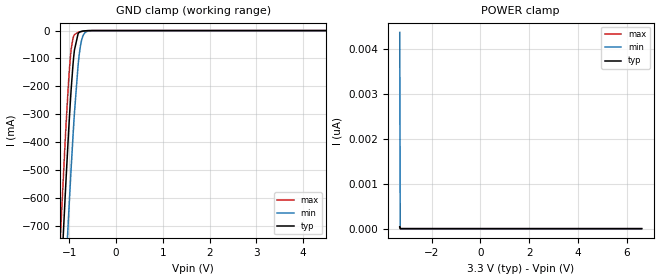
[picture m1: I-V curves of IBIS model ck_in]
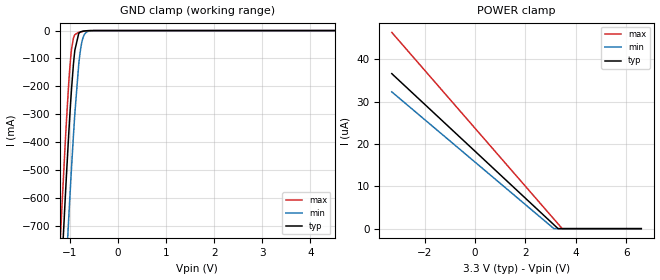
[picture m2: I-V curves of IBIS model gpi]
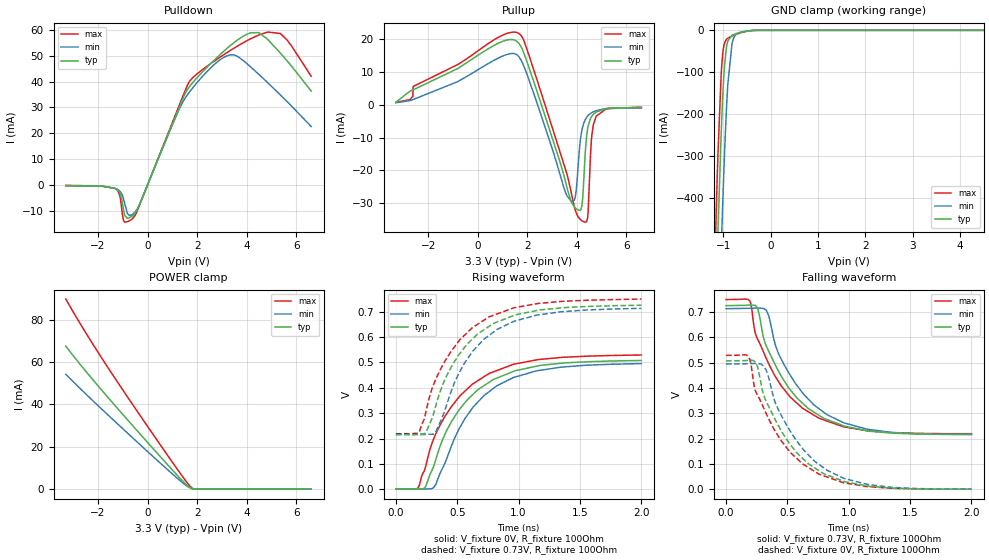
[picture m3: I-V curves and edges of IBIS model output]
|Texas Instruments Incorporated
| Marketing Part # : CDCDB803
| Voltage Range : 3.3V
| Package-type: QFN
| #pins/pkg drawing : 48-pin RSL
[IBIS Ver] 3.2
[File name] cdcdb803.ibs
[File Rev] 1.0
[Date] 07/02/2021
[Source]
| Texas Instruments Incorporated.
| 12500 TI Blvd
| Dallas, TX -75243
[Notes] Revision History:
| Rev 1.0: 07/02/2021
| - Initial version of the model
| - Model generated from simulations in TISPICE/SPECTRE
| - C_comp although listed in numerical order of value are
| obtained from varying PVT conditions. For PVT conditions for
| each specific value refer the buffer description under
| respective [Model]. IBIS model user is responsible for using
| appropriate C_comp to simulate for Signal Integrity.
| - Warnings regarding combined Non-monotonicity of various models have been
| reviewed and considered minor and can be ignored.
[Disclaimer]
| This model is designed as an aid for customers of Texas Instruments.
| TI and its licensors and suppliers make no warranties, either expressed
| or implied, with respect to this model, including the warranties of
| merchantability or fitness for a particular purpose. The model is
| provided solely on an "as is" basis. The entire risk as to its quality
| and performance is with the customer.
| This model is subject to change without notice. Texas Instruments
| Incorporated is not responsible for updating this model.
[Copyright]
(C) Copyright 2021 Texas Instruments Incorporated. All rights reserved.
| Component1 CDCDB803 (per package)
[Component] CDCDB803
[Manufacturer] Texas Instruments Incorporated
[Package] |48 QFN
| variable typ min max
R_pkg 0.111 0.052 0.169
L_pkg 2.02nH 1.12nH 2.9nH
C_pkg 0.163pF 0.062pF 0.264pF
| pin number (pin name) mapping to model name
[Pin] signal_name model_name R_pin L_pin C_pin
1   CLK_IN   ck_in   NA   NA   NA
2   CLK_INz   ck_in   NA   NA   NA
3   CK0P   output   NA   NA   NA
4   CK0N   output   NA   NA   NA
5   CK1P   output   NA   NA   NA
6   CK1N   output   NA   NA   NA
7   CK2P   output   NA   NA   NA
8   CK2N   output   NA   NA   NA
9   CK3P   output   NA   NA   NA
10   CK3N   output   NA   NA   NA
11   CK4P   output   NA   NA   NA
12   CK4N   output   NA   NA   NA
13   CK5P   output   NA   NA   NA
14   CK5N   output   NA   NA   NA
15   CK6P   output   NA   NA   NA
16   CK6N   output   NA   NA   NA
17   CK7P   output   NA   NA   NA
18   CK7N   output   NA   NA   NA
19   POWERGD_POWERDNz   gpi   NA   NA   NA
20   OE0B   gpi   NA   NA   NA
21   OE1B   gpi   NA   NA   NA
22   OE2B   gpi   NA   NA   NA
23   OE3B   gpi   NA   NA   NA
24   OE4B   gpi   NA   NA   NA
25   OE5B   gpi   NA   NA   NA
26   OE6B   gpi   NA   NA   NA
27   OE7B   gpi   NA   NA   NA
28   SMB_WRTLOCK   gpi   NA   NA   NA
29   VDD   POWER   NA   NA   NA
30   VDDR   POWER   NA   NA   NA
31   VDDA   POWER   NA   NA   NA
32   SMBDAT   smbdat   NA   NA   NA
33   SMBCLK   smbclk   NA   NA   NA
34   SADR0   strap_in   NA   NA   NA
35   SADR1   strap_in   NA   NA   NA
[Diff Pin]   inv_pin   vdiff   tdelay_typ  tdelay_min  tdelay_max
1   2   10m   NA   NA   NA
3   4   NA   NA   NA   NA
5   6   NA   NA   NA   NA
7   8   NA   NA   NA   NA
9   10   NA   NA   NA   NA
11   12   NA   NA   NA   NA
13   14   NA   NA   NA   NA
15   16   NA   NA   NA   NA
17   18   NA   NA   NA   NA
| Use Differential pin definition for differential I/Os
|[Diff Pin] inv_pin vdiff tdelay_typ tdelay_min tdelay_max
|3 4 200mV NA NA NA
|15 16 NA NA NA NA
|***** end of component 1 definition
| Models and submodels in the file (6): ck_in (Input), gpi (Input), output (Output), smbclk (Input), smbdat (I/O_open_drain), strap_in (Input)
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| Model Selectors
|***Modify the following as it applies to a speciic model with multiple ****
|*** powver supply options or driver programmability *********
| Model1
|IBIS Model File - Generated by SIMDE
| http://www.iometh.com/Product/SIMDE
[Model]   ck_in
Model_type   Input
Vinl = 0.66
Vinh = 2.64
|   typ   min   max
C_comp   1.16pF   1.09pF   1.19pF
[Voltage Range]   3.3   3.135   3.465
[Temperature Range]   27   125   -40
[Power Clamp Reference]   3.3   3.135   3.465
[GND Clamp Reference]   0   0   0
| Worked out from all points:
|   GND clamp passes 1 mA (typ) near -0.68 V on its own axis
[GND Clamp]
|   Voltage   I(typ)   I(min)   I(max)
-3.3V     -9.039A    -9.284A    -8.888A
-1.191V   -935.5mA   -1.251A    -732mA
-1.162V   -831.2mA   -1.146A    -628.1mA
-1.092V   -595.1mA   -906.9mA   -396mA
-1.023V   -374.9mA   -677.1mA   -191.4mA
-973.5mV  -234.8mA   -521.5mA   -82.42mA
-894.3mV  -70.11mA   -296.5mA   -14.46mA
-815.1mV  -10.89mA   -123.3mA   -6.064mA
-765.6mV  -4.002mA   -55.99mA   -4.283mA
-716.1mV  -1.883mA   -21.3mA    -2.535mA
-557.7mV  -94.7uA    -711uA     -73.04uA
6.6V      0A         0A         0A
[POWER Clamp]
|   Voltage   I(typ)   I(min)   I(max)
-3.3V     45.09pA    4.378nA    27.16pA
-3.28V    0A         0A         0A
-3.27V    0A         0A         0A
6.6V      0A         0A         0A
[Model]   gpi
Model_type   Input
Vinl = 1.2
Vinh = 1.6
|   typ   min   max
C_comp   0.852pF   0.8pF   0.9pF
[Voltage Range]   3.3   3.135   3.465
[Temperature Range]   27   125   -40
[Power Clamp Reference]   3.3   3.135   3.465
[GND Clamp Reference]   0   0   0
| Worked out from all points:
|   GND clamp passes 1 mA (typ) near -0.67 V on its own axis
[GND Clamp]
|   Voltage   I(typ)   I(min)   I(max)
-3.3V     -9.039A    -9.284A    -8.888A
-1.191V   -935.6mA   -1.251A    -732.1mA
-1.162V   -831.3mA   -1.146A    -628.1mA
-1.092V   -595.2mA   -907mA     -396.1mA
-1.023V   -375mA     -677.2mA   -191.6mA
-973.5mV  -235mA     -521.6mA   -82.67mA
-894.3mV  -70.36mA   -296.7mA   -14.69mA
-815.1mV  -11.07mA   -123.5mA   -6.196mA
-765.6mV  -4.101mA   -56.27mA   -4.378mA
-716.1mV  -1.934mA   -21.53mA   -2.594mA
-557.7mV  -100.1uA   -740.4uA   -78.62uA
6.6V      0A         0A         0A
[POWER Clamp]
|   Voltage   I(typ)   I(min)   I(max)
-3.3V     36.61uA    32.31uA    46.35uA
3.125V    960nA      39.57nA    2.319uA
3.293V    26nA       0A         1.165uA
3.462V    0A         0A         11.68nA
6.6V      0A         0A         0A
[Model]   output
Model_type   Output
Polarity   Non-Inverting
Vmeas = 0.365
Vref = 0
Cref = 2pF
Rref = 100000
|   typ   min   max
C_comp   4pF   3.5pF   4.5pF
[Voltage Range]   3.3   3.135   3.465
[Temperature Range]   27   125   -40
[Pullup Reference]   3.3   3.135   3.465
[Pulldown Reference]   0   -0   0
[Power Clamp Reference]   3.3   3.135   3.465
[GND Clamp Reference]   0   0   0
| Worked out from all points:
|   slope of the pulldown table from 0 to 0.495 V, typ, clamps not added: 42.1 ohm
|   GND clamp passes 1 mA (typ) near -0.44 V on its own axis
|   falling waveform, V_fixture 0.73V, R_fixture 100Ohm: 20-80 % time 377ps typ, 384ps min, 383ps max; typ from 0.725 V to 0.217 V
|   rising waveform, V_fixture 0V, R_fixture 100Ohm: 20-80 % time 396ps typ, 395ps min, 402ps max; typ from 0.001 V to 0.508 V
|   rising waveform, V_fixture 0.73V, R_fixture 100Ohm: 20-80 % time 382ps typ, 377ps min, 390ps max; typ from 0.217 V to 0.725 V
|   falling waveform, V_fixture 0V, R_fixture 100Ohm: 20-80 % time 378ps typ, 384ps min, 386ps max; typ from 0.507 V to 0.001 V
[Pulldown]
|   Voltage   I(typ)   I(min)   I(max)
-3.3V     -318.6uA   -393.1uA   -273.4uA
-1.31V    -1.398mA   -1.371mA   -1.435mA
-1.122V   -3.194mA   -2.494mA   -4.283mA
-973.5mV  -9.578mA   -5.349mA   -13.87mA
-815.1mV  -13.03mA   -11.21mA   -14.32mA
-636.9mV  -12.23mA   -11.62mA   -13.37mA
-379.5mV  -8.892mA   -8.671mA   -9.227mA
1.68V     37.96mA    35.85mA    39.95mA
3.244V    53.25mA    50.17mA    51.53mA
4.481V    59.02mA    42.89mA    58.09mA
5.353V    51.13mA    34.87mA    58.68mA
6.6V      36.35mA    22.57mA    42.09mA
[GND Clamp]
|   Voltage   I(typ)   I(min)   I(max)
-3.3V     -10.93A    -11.17A    -10.79A
-1.211V   -881.9mA   -1.2A      -686.4mA
-1.132V   -556.2mA   -867.4mA   -367.4mA
-1.112V   -480.1mA   -787.6mA   -296.1mA
-1.033V   -214.5mA   -487.9mA   -84.47mA
-1.013V   -162.9mA   -419.7mA   -57.48mA
-973.5mV  -85.09mA   -295mA     -30.33mA
-904.2mV  -25.82mA   -129mA     -18.86mA
-815.1mV  -11.68mA   -31.98mA   -13.66mA
-785.4mV  -10.14mA   -20.14mA   -12.18mA
-320.1mV  -99.39uA   -119.7uA   -85.22uA
6.6V      0A         0A         0A
[Pullup]
|   Voltage   I(typ)   I(min)   I(max)
-3.3V     815.4uA    650uA      792.1uA
848.1mV   18.92mA    14.39mA    20.72mA
1.65V     18.91mA    14.82mA    21.89mA
3.759V    -29.34mA   -29.32mA   -26.28mA
3.957V    -31.62mA   -27.07mA   -32.62mA
4.165V    -31.9mA    -9.367mA   -35.19mA
4.234V    -28.48mA   -6.653mA   -35.54mA
4.333V    -14.99mA   -4.554mA   -35.85mA
4.452V    -6.575mA   -3.241mA   -32.96mA
4.6V      -3.505mA   -2.356mA   -9.462mA
4.769V    -2.234mA   -1.788mA   -3.599mA
6.6V      -765.3uA   -936uA     -660uA
[POWER Clamp]
|   Voltage   I(typ)   I(min)   I(max)
-3.3V     67.46mA    54.22mA    89.73mA
-2.28V    52.65mA    42.55mA    69.77mA
-1.221V   38.21mA    30.92mA    50.67mA
1.175V    6.833mA    5.39mA     9.808mA
1.601V    1.727mA    1.368mA    2.963mA
1.789V    238.8uA    261.4uA    521.2uA
1.977V    4.57uA     9.613uA    7.6uA
6.6V      0A         0A         0A
[Ramp]
R_load = 100
|   typ   min   max
dV/dt_r   0.303987/3.95814e-10   0.296571/3.95271e-10   0.316807/4.01973e-10
dV/dt_f   0.304714/3.77209e-10   0.297744/3.83928e-10   0.317433/3.83478e-10
[Falling Waveform]
V_fixture = 0.73V
V_fixture_min = 0.72V
V_fixture_max = 0.75V
R_fixture = 100Ohm
C_fixture = 0F
|   Time   V(typ)   V(min)   V(max)
0s        725.2mV    713.2mV    749.2mV
190.9ps   727.4mV    714.7mV    745.7mV
237.4ps   726.4mV    715.4mV    617.5mV
258.9ps   714mV      715.5mV    591.4mV
326.6ps   567.8mV    708.4mV    518.1mV
449.8ps   447.3mV    513.6mV    409.1mV
629.2ps   337.7mV    377.4mV    318.8mV
757.1ps   292.6mV    318.7mV    281.1mV
1.146ns   232.2mV    238.1mV    231.9mV
2ns       217.4mV    217mV      220.1mV
[Rising Waveform]
V_fixture = 0V
V_fixture_min = 0V
V_fixture_max = 0V
R_fixture = 100Ohm
C_fixture = 0F
|   Time   V(typ)   V(min)   V(max)
0s        1.066mV    1.044mV    1.166mV
178.4ps   1.408mV    1.066mV    4.711mV
240.1ps   9.264mV    1.576mV    86.72mV
304.2ps   87.01mV    5.2mV      194.8mV
378.6ps   194.2mV    82.33mV    269.7mV
511.2ps   311.2mV    235.5mV    361.9mV
629.2ps   374.8mV    324.2mV    416.3mV
757.1ps   421mV      384mV      456mV
1.146ns   485.3mV    467mV      510mV
2ns       507.7mV    495.3mV    529.2mV
[Rising Waveform]
V_fixture = 0.73V
V_fixture_min = 0.72V
V_fixture_max = 0.75V
R_fixture = 100Ohm
C_fixture = 0F
|   Time   V(typ)   V(min)   V(max)
0s        216.6mV    215.6mV    219.4mV
190.9ps   217.8mV    215.7mV    228.2mV
240.1ps   221.8mV    216.5mV    295.6mV
326.6ps   332.2mV    228.7mV    435.9mV
413.4ps   447.6mV    333.3mV    516mV
513ps     530.4mV    457.8mV    584.1mV
629.2ps   594.8mV    546.1mV    639mV
757.1ps   641.5mV    605.9mV    678.9mV
1.146ns   704.1mV    686.1mV    731.2mV
2ns       725.2mV    712.8mV    749.5mV
[Falling Waveform]
|Gnd
V_fixture = 0V
V_fixture_min = 0V
V_fixture_max = 0V
R_fixture = 100Ohm
C_fixture = 0F
|   Time   V(typ)   V(min)   V(max)
0s        507.2mV    494.8mV    528.9mV
178.4ps   509.4mV    496.3mV    526.1mV
201.1ps   510.2mV    496.7mV    499.3mV
240.1ps   501.9mV    497.4mV    388.6mV
304.2ps   376.3mV    487.8mV    324.1mV
402.5ps   273.8mV    340.3mV    228.2mV
475.7ps   211.1mV    269.6mV    176mV
757.1ps   74.24mV    98.95mV    60.57mV
1.146ns   14.41mV    20.39mV    11.9mV
2ns       1.212mV    1.363mV    1.222mV
